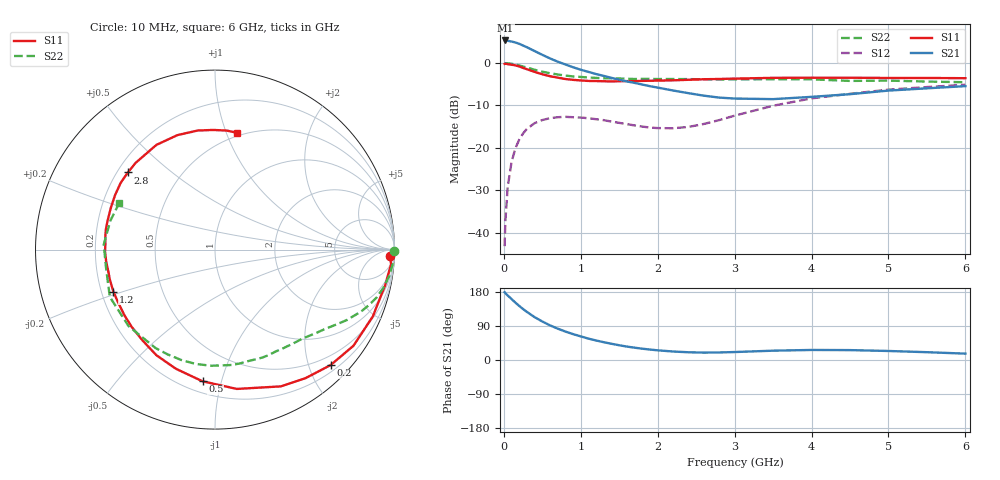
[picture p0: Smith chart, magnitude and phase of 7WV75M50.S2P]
! Infineon Technologies  Discrete & RF Semiconductors
! BFS17W
! Si NPN RF Bipolar Junction Transistor in SOT323
! VCE = 0.75 V  IC = 0.5 mA
! Common Emitter S-Parameters:  August  1999
# GHz  S  MA  R  50
!  f  S11  S21  S12  S22
! GHz  MAG  ANG  MAG  ANG  MAG  ANG  MAG  ANG
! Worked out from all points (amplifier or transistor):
!   36 points, 10 MHz to 6 GHz, reference 50 ohm
!   highest |S21| = 5.3 dB at 20 MHz (marker M1)
!   |S21| within 3 dB of that: start of sweep to 456.1 MHz
!   unconditionally stable (mu >= 1): 1.059 GHz to end of sweep
!   at 250 MHz: K = 0.27, MSG = 10.4 dB, |S12| = -16.6 dB
!   at 1.4 GHz: K = 1.28, MAG = 2.0 dB, |S12| = -13.8 dB
!   at 6 GHz: K = 1.14, MAG = -2.4 dB, |S12| = -5.1 dB
!   S11 on the Smith chart (normalised r, x): 10 MHz: 23, -38; 200 MHz: 0.32, -2.38; 500 MHz: 0.27, -0.87; 1.2 GHz: 0.25, -0.19; 2.8 GHz: 0.24, +0.36; 6 GHz: 0.47, +1.09
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0.01  0.9768 -2.2  1.829 178.9  0.0069 88.8  0.9999 -0.4
0.02  0.9843 -4.8  1.847 176.3  0.0137 89.0  0.9939 -1.8
0.05  0.9689 -11.7  1.83 170.3  0.0344 82.7  0.9936 -4.5
0.1  0.955 -22.9  1.794 161.0  0.0679 75.5  0.981 -8.8
0.15  0.9392 -34.8  1.749 151.4  0.0983 68.0  0.9613 -12.9
0.2  0.9103 -45.0  1.688 142.7  0.1249 62.1  0.9378 -16.7
0.3  0.8457 -64.3  1.536 126.9  0.1672 50.8  0.8846 -22.9
0.4  0.7858 -81.1  1.385 113.1  0.1952 41.5  0.833 -28.1
0.5  0.737 -95.4  1.25 101.6  0.2123 34.0  0.7913 -32.0
0.6  0.6987 -108.2  1.134 91.4  0.2237 28.4  0.7574 -35.6
0.8  0.6476 -128.5  0.962 75.1  0.2317 19.9  0.7118 -42.4
1.1  0.6148 -151.5  0.786 56.4  0.2232 12.5  0.6751 -52.2
1.2  0.6127 -157.5  0.741 51.5  0.2173 11.0  0.6675 -55.8
1.6  0.6128 -178.8  0.606 35.4  0.1901 10.7  0.6519 -69.8
2.2  0.6254 158.1  0.474 22.4  0.1701 26.8  0.6474 -92.0
2.8  0.6485 138.5  0.391 19.9  0.2121 44.4  0.6407 -114.3
3.5  0.6686 119.2  0.375 24.6  0.3133 47.4  0.6431 -138.5
4  0.6713 108.1  0.399 26.5  0.3828 42.8  0.6425 -155.8
4.5  0.6704 98.3  0.429 26.1  0.4334 37.0  0.6152 -170.9
5  0.6667 90.9  0.473 23.8  0.4854 31.5  0.6203 177.3
5.5  0.6665 84.4  0.503 20.6  0.5206 25.9  0.6047 164.5
6  0.6623 79.2  0.534 16.8  0.5545 20.7  0.5933 153.8
